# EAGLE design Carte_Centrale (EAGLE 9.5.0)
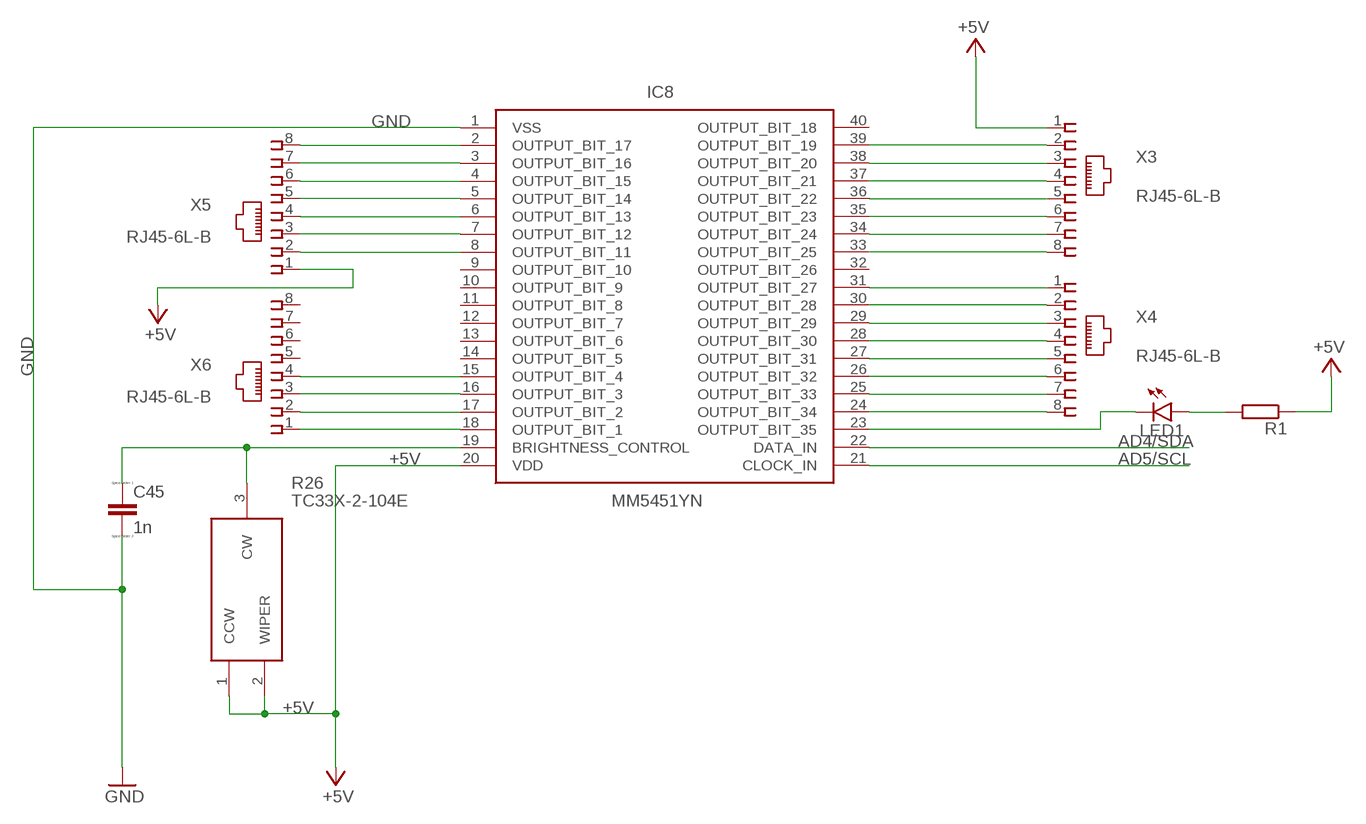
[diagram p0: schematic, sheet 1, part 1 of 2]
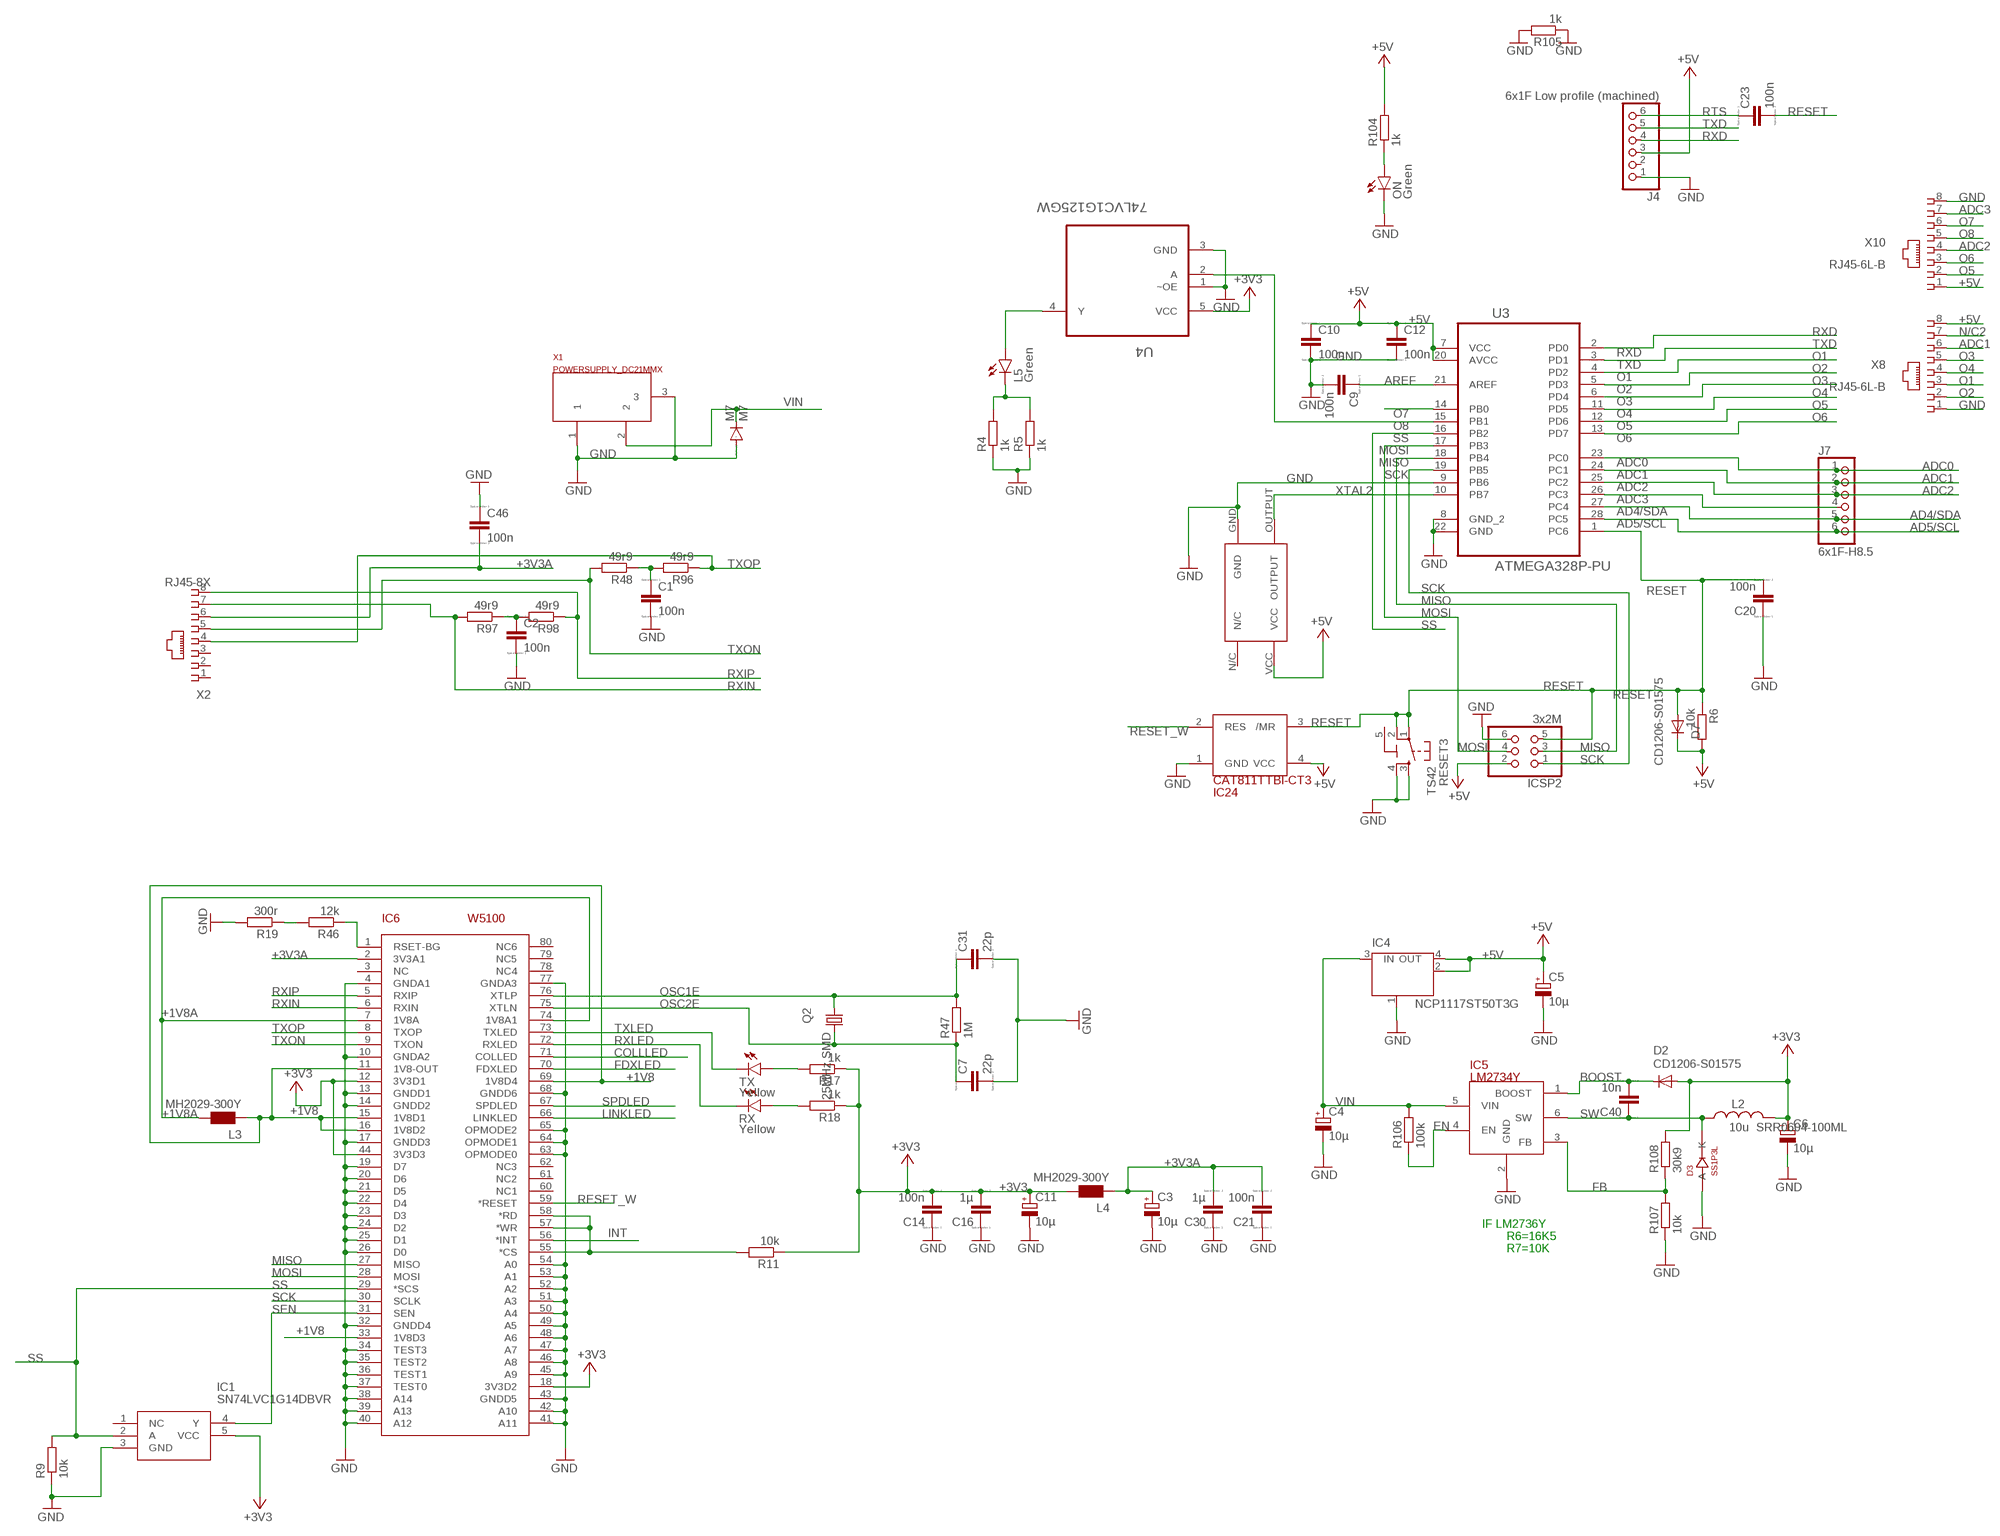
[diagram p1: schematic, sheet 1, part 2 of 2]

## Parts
C1  100n  CC2012  [C2012]
C2  100n  CC2012  [C2012]
C3  10µ  CPOL-EUE2-5  [E2-5]
C4  10µ  CPOL-EUE2-5  [E2-5]
C5  10µ  CPOL-EUE2-5  [E2-5]
C6  10µ  CPOL-EUE2-5  [E2-5]
C7  22p  CC2012  [C2012]
C9  100n  CC2012  [C2012]
C10  100n  CC2012  [C2012]
C11  10µ  CPOL-EUE2-5  [E2-5]
C12  100n  CC2012  [C2012]
C14  100n  CC2012  [C2012]
C16  1µ  CC2012  [C2012]
C20  100n  CC2012  [C2012]
C21  100n  CC2012  [C2012]
C23  100n  CC2012  [C2012]
C30  1µ  CC2012  [C2012]
C31  22p  CC2012  [C2012]
C40  10n  CC2012  [C2012]
C45  1n  CC2012  [C2012]
C46  100n  CC2012  [C2012]
D2  CD1206-S01575  DIODE-MINIMELF  [MINIMELF]
D3  SS1P3L  [DO220AAL]
D7  CD1206-S01575  DIODE-MINIMELF  [MINIMELF]
IC1  SN74LVC1G14DBVR  [SOT95P280X145-5N]
IC4  NCP1117ST50T3G  LINEAR_MC33269ST  [LINEAR_SOT223]
IC5  LM2734Y  LM2736Y  [SOT23-6]
IC6  W5100  [SQFP-S-10X10-80]
IC8  MM5451YN  [DIP1556W46P254L5207H635Q40N]
IC24  CAT811TTBI-CT3  STM812  [SOT143]
ICSP2  3x2M  PINHD-2X3  [2X03]
J4  6x1F Low profile (machined)  PINHD-1X6TH  [1X06-TH]
J7  6x1F-H8.5  PINHD-1X6  [1X06]
L2  10u SRR0604-100ML  L-USSRR0604  [SRR0604]
L3  MH2029-300Y  WE-CBF_0805  [0805]
L4  MH2029-300Y  WE-CBF_0805  [0805]
L5  Green  LEDCHIPLED_0805  [CHIPLED_0805]
LED1  LED5MM  [LED5MM]
M7  M7  1N4004  [DO41-10]
ON  Green  LEDCHIPLED_0805  [CHIPLED_0805]
Q2  25MHz SMD  CRYSTALHC49UP  [HC49UP]
R1  R-EU_0204/7  [0204/7]
R4  1k  R-EU_M0805  [M0805]
R5  1k  R-EU_M0805  [M0805]
R6  10k  R-EU_M0805  [M0805]
R9  10k  R-EU_M0805  [M0805]
R11  10k  R-EU_M0805  [M0805]
R17  1k  R-EU_M0805  [M0805]
R18  1k  R-EU_M0805  [M0805]
R19  300r  R-EU_M0805  [M0805]
R26  TC33X-2-104E  [TC33X-2]
R46  12k  R-EU_M0805  [M0805]
R47  1M  R-EU_M0805  [M0805]
R48  49r9  R-EU_M0805  [M0805]
R96  49r9  R-EU_M0805  [M0805]
R97  49r9  R-EU_M0805  [M0805]
R98  49r9  R-EU_M0805  [M0805]
R104  1k  R-EU_M0805  [M0805]
R105  1k  R-EU_M0805  [M0805]
R106  100k  R-EU_M0805  [M0805]
R107  10k  R-EU_M0805  [M0805]
R108  30k9  R-EU_M0805  [M0805]
RESET3  TS42  [TS42]
RX  Yellow  LEDCHIPLED_0805  [CHIPLED_0805]
TX  Yellow  LEDCHIPLED_0805  [CHIPLED_0805]
U3  ATMEGA328P-PU  [DIP254P762X457-28]
U4  74LVC1G125GW  [SOT65P210X110-5N]
U$1  NCT050C  [NCT050C_FOOTPRINT]
X1  POWERSUPPLY_DC21MMX  [POWERSUPPLY_DC-21MM]
X2  RJ45-8X  [RJ45-NO-SHIELD]
X3  RJ45-6L-B  [RJ45-NO-SHIELD]
X4  RJ45-6L-B  [RJ45-NO-SHIELD]
X5  RJ45-6L-B  [RJ45-NO-SHIELD]
X6  RJ45-6L-B  [RJ45-NO-SHIELD]
X8  RJ45-6L-B  [RJ45-NO-SHIELD]
X10  RJ45-6L-B  [RJ45-NO-SHIELD]

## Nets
+1V8 [power]: IC6.11(1V8-OUT) IC6.15(1V8D1) IC6.16(1V8D2) IC6.33(1V8D3) IC6.69(1V8D4) L3.1
+1V8A [power]: IC6.7(1V8A) IC6.74(1V8A1) L3.2
+3V3 [power]: C6.+ C11.+ C14.2 C16.2 D2.A IC1.5(VCC) IC6.12(3V3D1) IC6.18(3V3D2) IC6.44(3V3D3) L2.P$2 L4.2 R11.1 R17.1 R18.1 R108.2 U4.5(VCC)
+3V3A [power]: C3.+ C21.2 C30.2 C46.2 IC6.2(3V3A1) L4.1 X2.6
+5V [power]: C5.+ C10.1 C12.1 D7.C IC4.2(OUT) IC4.4(OUT) IC8.20(VDD) IC24.4(VCC) ICSP2.2 J4.3 R1.1 R6.2 R26.1(CCW) R26.2(WIPER) R104.2 U3.7(VCC) U3.20(AVCC) U$1.VCC X3.1 X5.1 X8.8 X10.1
AD4/SDA: IC8.22(DATA_IN) J7.5 U3.27(PC4)
AD5/SCL: IC8.21(CLOCK_IN) J7.6 U3.28(PC5)
ADC0: J7.1 U3.23(PC0)
ADC1: J7.2 U3.24(PC1) X8.6
ADC2: J7.3 U3.25(PC2) X10.4
ADC3: J7.4 U3.26(PC3) X10.7
AREF: C9.1 U3.21(AREF)
BOOST: C40.2 D2.C IC5.1(BOOST)
COLLLED: IC6.71(COLLED)
EN: IC5.4(EN) R106.1
FB: IC5.3(FB) R107.2 R108.1
FDXLED: IC6.70(FDXLED)
GND: C1.2 C2.2 C3.- C4.- C5.- C6.- C7.2 C9.2 C10.2 C11.- C12.2 C14.1 C16.1 C20.1 C21.1 C30.1 C31.2 C45.2 C46.1 D3.P$2(A) IC1.3(GND) IC4.1(GND/ADJ) IC5.2(GND) IC6.4(GNDA1) IC6.10(GNDA2) IC6.13(GNDD1) IC6.14(GNDD2) IC6.17(GNDD3) IC6.19(D7) IC6.20(D6) IC6.21(D5) IC6.22(D4) IC6.23(D3) IC6.24(D2) IC6.25(D1) IC6.26(D0) IC6.32(GNDD4) IC6.34(TEST3) IC6.35(TEST2) IC6.36(TEST1) IC6.37(TEST0) IC6.38(A14) IC6.39(A13) IC6.40(A12) IC6.41(A11) IC6.42(A10) IC6.43(GNDD5) IC6.45(A9) IC6.46(A8) IC6.47(A7) IC6.48(A6) IC6.49(A5) IC6.50(A4) IC6.51(A3) IC6.52(A2) IC6.53(A1) IC6.54(A0) IC6.63(OPMODE0) IC6.64(OPMODE1) IC6.65(OPMODE2) IC6.68(GNDD6) IC6.77(GNDA3) IC8.1(VSS) IC24.1(GND) ICSP2.6 J4.1 M7.A ON.C R4.1 R5.1 R9.1 R19.2 R105.1 R105.2 R107.1 RESET3.3 RESET3.4 U3.8(GND_2) U3.9(PB6) U3.22(GND) U4.1(~OE) U4.3(GND) U$1.GND X1.1 X1.3 X8.1 X10.8
INT: IC6.56(*INT)
LINKLED: IC6.66(LINKLED)
MISO: IC6.27(MISO) ICSP2.3 U3.18(PB4)
MOSI: IC6.28(MOSI) ICSP2.4 U3.17(PB3)
N$6: IC8.2(OUTPUT_BIT_17) X5.8
N$7: IC8.3(OUTPUT_BIT_16) X5.7
N$8: ON.A R104.1
N$9: R17.2 TX.A
N$10: C1.1 R48.1 R96.2
N$11: IC8.4(OUTPUT_BIT_15) X5.6
N$12: IC8.5(OUTPUT_BIT_14) X5.5
N$16: L5.A U4.4(Y)
N$17 [power]: C45.1 IC8.19(BRIGHTNESS_CONTROL) R26.3(CW)
N$20: IC8.6(OUTPUT_BIT_13) X5.4
N$21: IC8.7(OUTPUT_BIT_12) X5.3
N$22: R18.2 RX.A
N$23: IC8.8(OUTPUT_BIT_11) X5.2
N$25: LED1.A R1.2
N$29: C2.1 R97.1 R98.2
N$30: R19.1 R46.2
N$31: IC6.1(RSET-BG) R46.1
N$32: IC8.15(OUTPUT_BIT_4) X6.4
N$33: IC8.16(OUTPUT_BIT_3) X6.3
N$34: IC8.17(OUTPUT_BIT_2) X6.2
N$35: IC8.18(OUTPUT_BIT_1) X6.1
N$36: IC6.55(*CS) IC6.57(*WR) IC6.58(*RD) R11.2
N$38: IC8.39(OUTPUT_BIT_19) X3.2
N$39: IC8.38(OUTPUT_BIT_20) X3.3
N$40: IC8.37(OUTPUT_BIT_21) X3.4
N$41: IC8.36(OUTPUT_BIT_22) X3.5
N$42: IC8.35(OUTPUT_BIT_23) X3.6
N$43: IC8.34(OUTPUT_BIT_24) X3.7
N$44: IC8.33(OUTPUT_BIT_25) X3.8
N$45: IC8.31(OUTPUT_BIT_27) X4.1
N$46: IC8.30(OUTPUT_BIT_28) X4.2
N$47: IC8.29(OUTPUT_BIT_29) X4.3
N$48: IC8.28(OUTPUT_BIT_30) X4.4
N$49: IC8.27(OUTPUT_BIT_31) X4.5
N$50: IC8.26(OUTPUT_BIT_32) X4.6
N$51: IC8.25(OUTPUT_BIT_33) X4.7
N$52: IC8.24(OUTPUT_BIT_34) X4.8
N$54: L5.C R4.2 R5.2
N$55: IC8.23(OUTPUT_BIT_35) LED1.K(C)
N/C2: X8.7
O1: U3.4(PD2) X8.3
O2: U3.5(PD3) X8.2
O3: U3.6(PD4) X8.5
O4: U3.11(PD5) X8.4
O5: U3.12(PD6) X10.2
O6: U3.13(PD7) X10.3
O7: U3.14(PB0) X10.6
O8: U3.15(PB1) U4.2(A) X10.5
OSC1E: C31.1 IC6.76(XTLP) Q2.1 R47.2
OSC2E: C7.1 IC6.75(XTLN) Q2.2 R47.1
RESET: C20.2 C23.2 D7.A IC24.3(/MR) ICSP2.5 R6.1 RESET3.1 RESET3.2 U3.1(PC6)
RESET_W: IC6.59(*RESET) IC24.2(RES)
RTS: C23.1 J4.6
RXD: J4.4 U3.2(PD0)
RXIN: IC6.6(RXIN) R97.2 X2.7
RXIP: IC6.5(RXIP) R98.1 X2.8
RXLED: IC6.72(RXLED) RX.C
SCK: IC6.30(SCLK) ICSP2.1 U3.19(PB5)
SEN: IC1.4(Y) IC6.31(SEN)
SPDLED: IC6.67(SPDLED)
SS: IC1.2(A) IC6.29(*SCS) R9.2 U3.16(PB2)
SW [power]: C40.1 D3.P$1(K) IC5.6(SW) L2.P$1
TXD: J4.5 U3.3(PD1)
TXLED: IC6.73(TXLED) TX.C
TXON: IC6.9(TXON) R48.2 X2.5
TXOP: IC6.8(TXOP) R96.1 X2.4
VIN [VIN]: C4.+ IC4.3(IN) IC5.5(VIN) M7.C R106.2 X1.2
XTAL2: U3.10(PB7) U$1.OUTPUT
Unconnected: IC1.1(NC) IC6.3(NC) IC6.60(NC1) IC6.61(NC2) IC6.62(NC3) IC6.78(NC4) IC6.79(NC5) IC6.80(NC6) IC8.9(OUTPUT_BIT_10) IC8.10(OUTPUT_BIT_9) IC8.11(OUTPUT_BIT_8) IC8.12(OUTPUT_BIT_7) IC8.13(OUTPUT_BIT_6) IC8.14(OUTPUT_BIT_5) IC8.32(OUTPUT_BIT_26) IC8.40(OUTPUT_BIT_18) J4.2 U$1.N/C X2.1 X2.2 X2.3 X6.5 X6.6 X6.7 X6.8

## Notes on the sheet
- IF LM2736Y
- R6=16K5
- R7=10K

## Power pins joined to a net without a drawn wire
5-GND: RESET3.5(5-GND)

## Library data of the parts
C1 C2 C7 C9 C10 C12 C14 C16 C20 C21 C23 C30 C31 C40 C45 C46 = eagle-ltspice:C: CAPACITOR, European symbol; SPICEMODEL: NONE; SPICEPREFIX: C
C3-C6 C11 = rcl:CPOL-EU: POLARIZED CAPACITOR, European symbol; SPICEPREFIX: C
D2 D7 = diode:DIODE-: DIODE
D3 = SmartPrj:SS1P3L
IC1 = SN74LVC1G14DBVR:SN74LVC1G14DBVR: TEXAS INSTRUMENTS - SN74LVC1G14DBVR - IC, SCHMITT TRIGGER INVERTER, SMD Source: Datasheet; DESCRIPTION: TEXAS INSTRUMENTS - SN74LVC1G14DBVR - IC, SCHMITT TRIGGER INVERTER, SMD; HEIGHT: 1.45mm; MANUFACTURER_NAME: Texas Instruments; MANUFACTURER_PART_NUMBER: SN74LVC1G14DBVR; MOUSER_PART_NUMBER: 595-SN74LVC1G14DBVR; MOUSER_PRICE-STOCK: https://www.mouser.com/Search/Refine.aspx?Keyword=595-SN74LVC1G14DBVR
IC4 = SmartPrj:LINEAR_MC33269ST*: Adjustable Output Low Dropout Voltage Regulator 800 mA Source: http://www.onsemi.com/pub/Collateral/MC33269-D.PDF
IC5 = SmartPrj:LM2736Y
IC6 = SmartPrj:W5100
IC8 = SamacSys_Parts:MM5451YN: MM5451YN, LED Driver, 5-Digits, 5 V, 9 V, 40-Pin PDIP Source: Datasheet; DESCRIPTION: MM5451YN, LED Driver, 5-Digits, 5 V, 9 V, 40-Pin PDIP; HEIGHT: 6.35mm; MANUFACTURER_NAME: Micrel; MANUFACTURER_PART_NUMBER: MM5451YN; MOUSER_PART_NUMBER: 998-MM5451YN; MOUSER_PRICE-STOCK: https://www.mouser.com/Search/Refine.aspx?Keyword=998-MM5451YN
IC24 = SmartPrj:STM812
ICSP2 = SmartPrj:PINHD-2X3: PIN HEADER
J4 J7 = SmartPrj:PINHD-1X6: PIN HEADER
L2 = SmartPrj:L-US: INDUCTOR, American symbol
L3 L4 = wuerth-elektronik:WE-CBF: SMD EMI Suppression Ferrite Beads
L5 LED1 ON RX TX = led:LED: LED
M7 = diode:1N4004: DIODE
Q2 = crystal:CRYSTAL: CRYSTAL; OC_FARNELL: unknown; OC_NEWARK: unknown
R1 R4-R6 R9 R11 R17-R19 R46-R48 R96-R98 R104-R108 = rcl:R-EU_: RESISTOR, European symbol; SPICEPREFIX: R
R26 = TC33X-2-104E:TC33X-2-104E: Cermet 3mm SMT trimmer,0.1W 100k Bourns TC33 Series SMD Cermet Trimmer Resistor with Solder Pad Terminations, 100k +/-25% 1/10W +/-250ppm/C Top Adjust Source: Datasheet; ALLIED_NUMBER: 70155236; ALLIED_PRICE-STOCK: https://www.alliedelec.com/bourns-tc33x-2-104e/70155236/; DESCRIPTION: Cermet 3mm SMT trimmer,0.1W 100k Bourns TC33 Series SMD Cermet Trimmer Resistor with Solder Pad Terminations, 100k +/-25% 1/10W +/-250ppm/C Top Adjust; HEIGHT: mm; MANUFACTURER_NAME: Bourns; MANUFACTURER_PART_NUMBER: TC33X-2-104E; MOUSER_PART_NUMBER: 652-TC33X-2-104E; MOUSER_PRICE-STOCK: https://www.mouser.com/Search/Refine.aspx?Keyword=652-TC33X-2-104E; RS_PART_NUMBER: 4617258P; RS_PRICE-STOCK: http://uk.rs-online.com/web/p/products/4617258P
RESET3 = SmartPrj:TS42: TS42 Dongnan Electronics Tact switch VDC 12V - 50mA
U3 = Farnell_ATMEGA328PU:ATMEGA328P-PU: 8-bit Microcontroller with In-System Programmable Flash; MPN: ATMEGA328P-PU; OC_FARNELL: 1715487; OC_NEWARK: 68T2944; PACKAGE: PDIP-28; SUPPLIER: Atmel
U4 = Farnell_74LVC1G125GW:74LVC1G125GW: Bus buffer/line driver 3-state; MPN: 74LVC1G125GW; OC_FARNELL: 1631685; OC_NEWARK: 03P2776; PACKAGE: SOT-5; SUPPLIER: NXP
U$1 = NCT050C:NCT050C
X1 = SmartPrj:POWERSUPPLY_DC21MM
X2 = con-tycoelectronics:RJ45: CORCOM Modular RJ Jacks No Shield Source: www.tycoelectronics.com .. ENG_DS_1654001_1099_RJ_L_0507.pdf; MPN: RJ45-8X; OC_FARNELL: unknown; OC_NEWARK: 16R6101
X3-X6 X8 X10 = con-tycoelectronics:RJ45: CORCOM Modular RJ Jacks No Shield Source: www.tycoelectronics.com .. ENG_DS_1654001_1099_RJ_L_0507.pdf; MPN: RJ45-6L-B; OC_FARNELL: unknown; OC_NEWARK: 16R6090

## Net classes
0 default: width 0.152 mm, drill 0.61 mm, clearance 0.152 mm
1 power: width 0.152 mm, drill 0.61 mm, clearance 0.152 mm
2 VIN: width 0.61 mm, drill 0.61 mm, clearance 0.254 mm

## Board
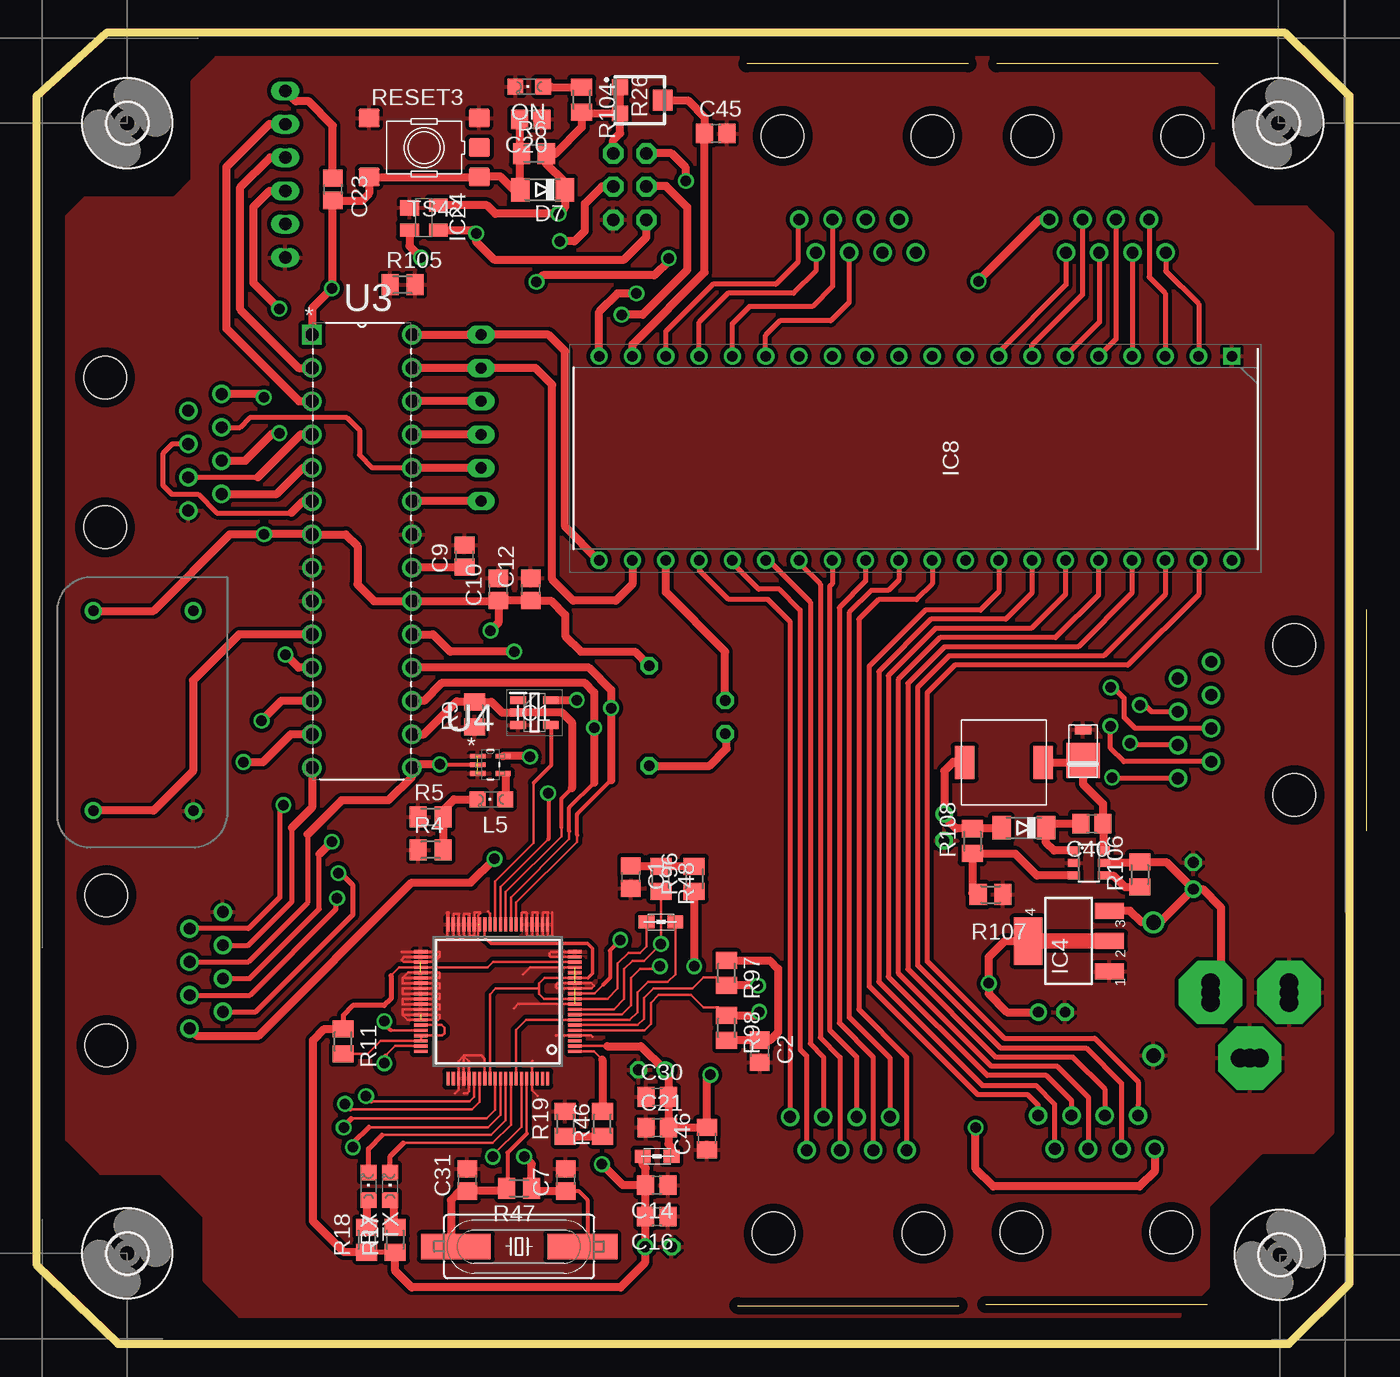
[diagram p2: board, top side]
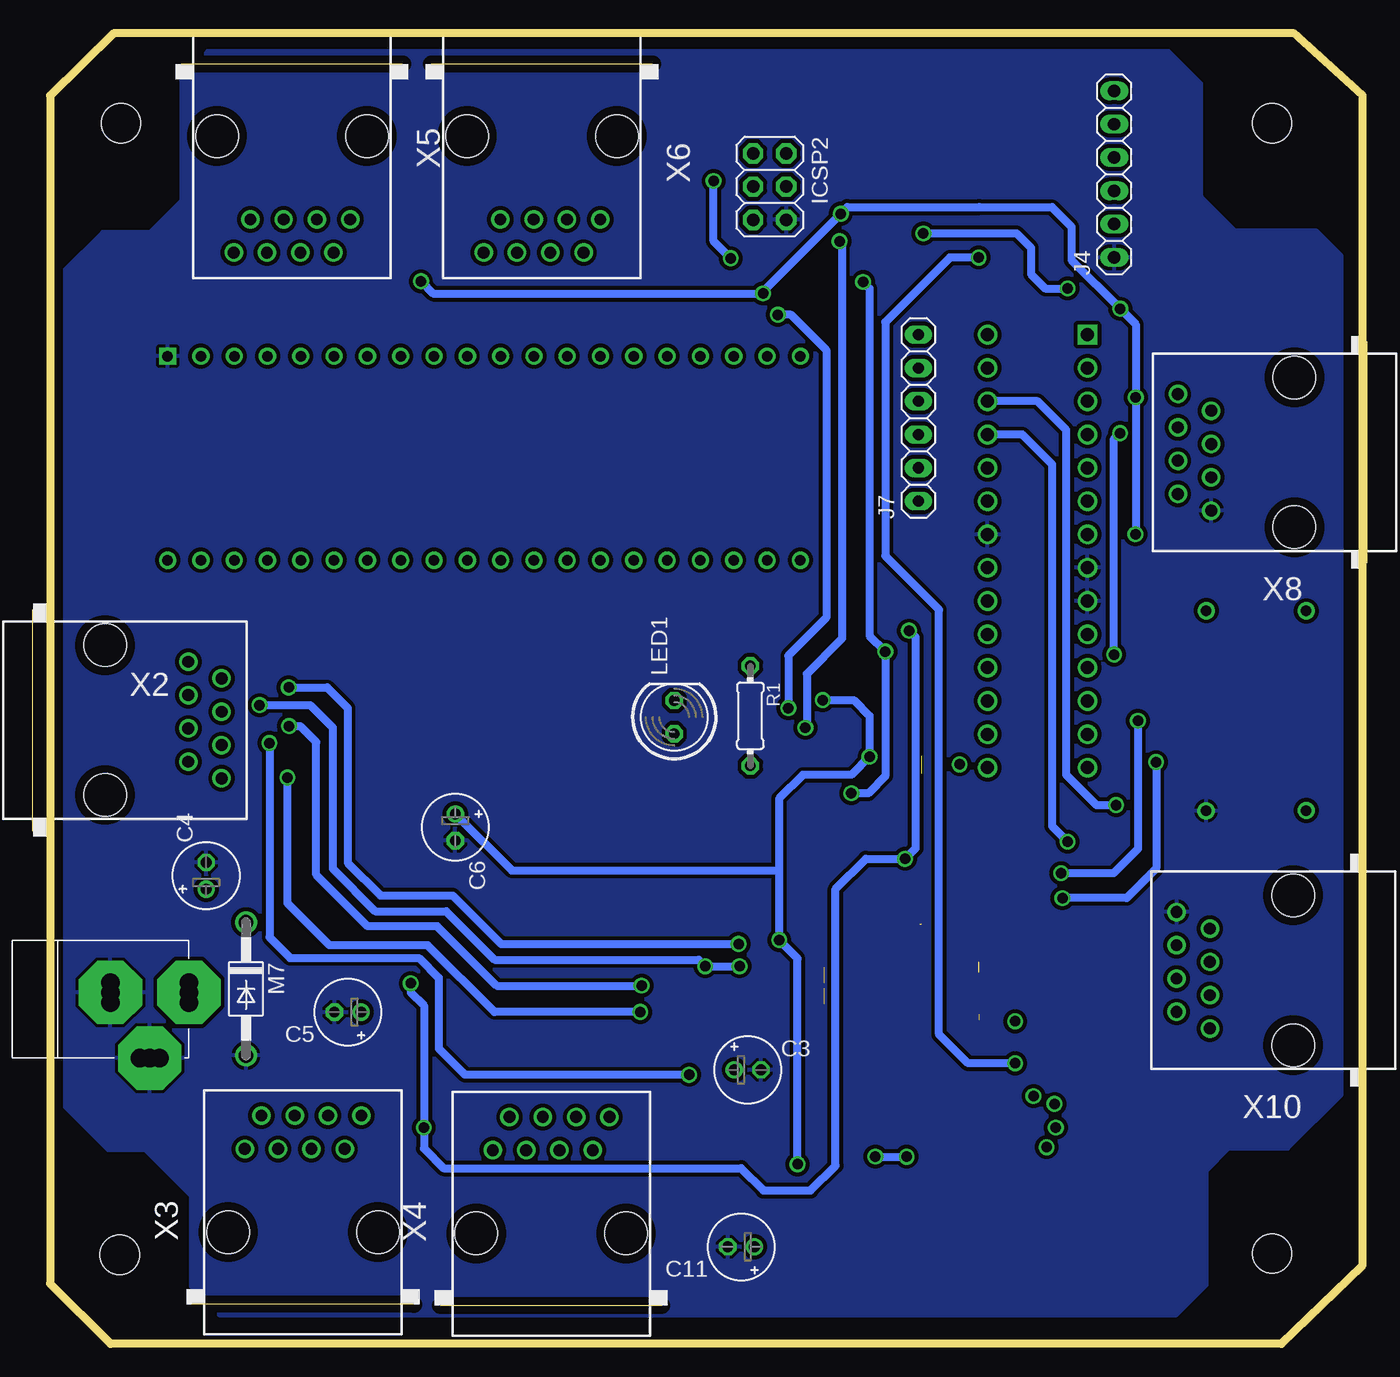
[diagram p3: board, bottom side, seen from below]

Size 101.74 x 100 mm. Coordinates in mm from the lower left corner, seen from the top.
Outline: 0.31,95.2 5.61,100 95.51,100 100.41,95.2 100.41,4.6 95.81,0 6.51,0 0.31,6 0.31,95.2
Copper layers (1*16): Top 0.035mm / dielectric 1.5mm / Bottom 0.035mm
Design rules "ArduinoETH *": minimum track width 0.2mm, minimum drill 0.8mm, track to track 0.3mm, track to pad 0.3mm, pad to pad 0.2mm, via to via 0.2mm, smd to smd 0.3mm, copper to edge 25mil, drill to drill 10mil, minimum pad ring 10mil, minimum via ring 8mil, stop-mask expansion 1mil, vias tented up to drill 30mil, thermal gap 10mil

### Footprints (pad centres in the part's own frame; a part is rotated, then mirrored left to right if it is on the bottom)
C2012 = smd 1.3 x 1.5: 1 -0.85,0; 2 0.85,0
E2-5 = drill 0.813 pad 1.27: + -1.016,0 | drill 0.813 pad 1.27 octagon: - 1.016,0
MINIMELF = smd 1.4 x 1.8: A 1.7,0; C -1.7,0
DO220AAL = smd 2.667 x 2.54: P$1 -0.7,0 | smd 0.762 x 1.27: P$2 1.65,0
SOT95P280X145-5N = smd 1.2 x 0.6: 1 -1.25,0.95; 2 -1.25,0; 3 -1.25,-0.95; 4 1.25,-0.95; 5 1.25,0.95
LINEAR_SOT223 = smd 1.219 x 2.235: 1 -2.311,-3.099; 2 0,-3.099; 3 2.311,-3.099 | smd 3.6 x 2.2: 4 0,3.099
SOT23-6 = smd 0.6 x 0.9: 1 -0.95,-1.15; 2 0,-1.15; 3 0.95,-1.15; 4 0.95,1.15; 5 0,1.15; 6 -0.95,1.15
SQFP-S-10X10-80 = smd 0.241 x 1.041: 1 -3.8,-5.879; 2 -3.4,-5.879; 3 -3,-5.879; 4 -2.6,-5.879; 5 -2.2,-5.879; 6 -1.8,-5.879; 7 -1.4,-5.879; 8 -1,-5.879; 9 -0.6,-5.879; 10 -0.2,-5.879; 11 0.2,-5.879; 12 0.6,-5.879; 13 1,-5.879; 14 1.4,-5.879; 15 1.8,-5.879; 16 2.2,-5.879; 17 2.6,-5.879; 18 3,-5.879; 19 3.4,-5.879; 20 3.8,-5.879; 41 3.8,5.879; 42 3.4,5.879; 43 3,5.879; 44 2.6,5.879; 45 2.2,5.879; 46 1.8,5.879; 47 1.4,5.879; 48 1,5.879; 49 0.6,5.879; 50 0.2,5.879; 51 -0.2,5.879; 52 -0.6,5.879; 53 -1,5.879; 54 -1.4,5.879; 55 -1.8,5.879; 56 -2.2,5.879; 57 -2.6,5.879; 58 -3,5.879; 59 -3.4,5.879; 60 -3.8,5.879 | smd 1.041 x 0.241: 21 5.879,-3.8; 22 5.879,-3.4; 23 5.879,-3; 24 5.879,-2.6; 25 5.879,-2.2; 26 5.879,-1.8; 27 5.879,-1.4; 28 5.879,-1; 29 5.879,-0.6; 30 5.879,-0.2; 31 5.879,0.2; 32 5.879,0.6; 33 5.879,1; 34 5.879,1.4; 35 5.879,1.8; 36 5.879,2.2; 37 5.879,2.6; 38 5.879,3; 39 5.879,3.4; 40 5.879,3.8; 61 -5.879,3.8; 62 -5.879,3.4; 63 -5.879,3; 64 -5.879,2.6; 65 -5.879,2.2; 66 -5.879,1.8; 67 -5.879,1.4; 68 -5.879,1; 69 -5.879,0.6; 70 -5.879,0.2; 71 -5.879,-0.2; 72 -5.879,-0.6; 73 -5.879,-1; 74 -5.879,-1.4; 75 -5.879,-1.8; 76 -5.879,-2.2; 77 -5.879,-2.6; 78 -5.879,-3; 79 -5.879,-3.4; 80 -5.879,-3.8
DIP1556W46P254L5207H635Q40N = drill 0.8 pad 1.057 square: 1 -7.779,24.13 | drill 0.8 pad 1.057: 2 -7.779,21.59; 3 -7.779,19.05; 4 -7.779,16.51; 5 -7.779,13.97; 6 -7.779,11.43; 7 -7.779,8.89; 8 -7.779,6.35; 9 -7.779,3.81; 10 -7.779,1.27; 11 -7.779,-1.27; 12 -7.779,-3.81; 13 -7.779,-6.35; 14 -7.779,-8.89; 15 -7.779,-11.43; 16 -7.779,-13.97; 17 -7.779,-16.51; 18 -7.779,-19.05; 19 -7.779,-21.59; 20 -7.779,-24.13; 21 7.779,-24.13; 22 7.779,-21.59; 23 7.779,-19.05; 24 7.779,-16.51; 25 7.779,-13.97; 26 7.779,-11.43; 27 7.779,-8.89; 28 7.779,-6.35; 29 7.779,-3.81; 30 7.779,-1.27; 31 7.779,1.27; 32 7.779,3.81; 33 7.779,6.35; 34 7.779,8.89; 35 7.779,11.43; 36 7.779,13.97; 37 7.779,16.51; 38 7.779,19.05; 39 7.779,21.59; 40 7.779,24.13
SOT143 = smd 1.2 x 1.44: 1 -0.75,-1.1 | smd 1 x 1.44: 2 0.95,-1.1; 3 0.95,1.1; 4 -0.95,1.1
2X03 = drill 0.95 pad 1.55 octagon: 1 -2.54,-1.27; 2 -2.54,1.27; 3 0,-1.27; 4 0,1.27; 5 2.54,-1.27; 6 2.54,1.27
1X06-TH = drill 0.95 pad 1.422 long: 1 -6.35,0; 2 -3.81,0; 3 -1.27,0; 4 1.27,0; 5 3.81,0; 6 6.35,0
1X06 = drill 0.85 pad 1.422 long: 1 -6.35,0; 2 -3.81,0; 3 -1.27,0; 4 1.27,0; 5 3.81,0; 6 6.35,0
SRR0604 = smd 1.5 x 2.5: P$1 3,0; P$2 -3,0
0805 = smd 1.2 x 1: 1 -1.1,0; 2 1.1,0
CHIPLED_0805 = smd 1.2 x 1.2: A 0,-1.05; C 0,1.05
LED5MM = drill 0.813 octagon: A -1.27,0; K 1.27,0
DO41-10 = drill 1.118: A 5.08,0; C -5.08,0
HC49UP = smd 5.334 x 1.93: 1 -4.826,0; 2 4.826,0
0204/7 = drill 0.813 octagon: 1 -3.81,0; 2 3.81,0
M0805 = smd 1.3 x 1.6: 1 -0.95,0; 2 0.95,0
TC33X-2 = smd 1.2 x 1.2: 1 -1,-1.625; 2 1,-1.625 | smd 1.6 x 1.5: 3 0,1.625
TS42 = smd 1.6 x 1.4: 1 -4.2,2.25; 2 4.2,2.25; 3 -4.2,-2.25; 4 4.2,-2.25; 5 -4.2,0
DIP254P762X457-28 = drill 0.991 square: 1 -7.62,33.02 | drill 0.991: 2 -7.62,30.48; 3 -7.62,27.94; 4 -7.62,25.4; 5 -7.62,22.86; 6 -7.62,20.32; 7 -7.62,17.78; 8 -7.62,15.24; 9 -7.62,12.7; 10 -7.62,10.16; 11 -7.62,7.62; 12 -7.62,5.08; 13 -7.62,2.54; 14 -7.62,0; 15 0,0; 16 0,2.54; 17 0,5.08; 18 0,7.62; 19 0,10.16; 20 0,12.7; 21 0,15.24; 22 0,17.78; 23 0,20.32; 24 0,22.86; 25 0,25.4; 26 0,27.94; 27 0,30.48; 28 0,33.02
SOT65P210X110-5N = smd 1.168 x 0.356: 1 -0.965,0.66; 2 -0.965,0; 3 -0.965,-0.66; 4 0.965,-0.66; 5 0.965,0.66
NCT050C_FOOTPRINT = drill 0.8: GND -7.44,3.74; N/C 7.82,3.73; OUTPUT -7.42,-3.89; VCC 7.81,-3.9
3,0 = hole 3: 0,0
POWERSUPPLY_DC-21MM = drill 1.4 pad 4.826 octagon: 1 -5.08,-3.353; 2 -0.076,-6.35; 3 -0.076,-0.356 | drill 1.4: 4 -5.08,-4.115; 5 -5.08,-2.591; 6 -0.838,-0.356; 7 0.686,-0.356; 8 -0.838,-6.35; 9 0.686,-6.35
RJ45-NO-SHIELD = drill 0.9 pad 1.4: 1 -4.445,6.35; 2 -3.175,8.89; 3 -1.905,6.35; 4 -0.635,8.89; 5 0.635,6.35; 6 1.905,8.89; 7 3.175,6.35; 8 4.445,8.89 | hole 3.251: -5.715,0; 5.715,0

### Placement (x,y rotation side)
C1  45.62,35.6 270 top
C2  55.46,22.32 270 top
C3  47.21,20.9 0 bottom
C4  88.51,35.7 90 bottom
C5  77.71,25.3 180 bottom
C6  69.51,39.4 270 bottom
C7  40.65,12.51 90 top
C9  32.93,60.08 90 top
C10  35.52,57.54 90 top
C11  47.71,7.4 180 bottom
C12  37.97,57.54 90 top
C14  47.6,12.11 180 top
C16  47.6,9.72 180 top
C20  37.99,93.39 180 top
C21  47.62,16.5 0 top
C23  22.88,88.06 270 top
C30  47.62,18.84 0 top
C31  33.14,12.51 90 top
C40  80.77,39.68 180 top
C45  52.09,92.32 0 top
C46  51.42,15.66 90 top
D2  75.59,39.36 180 top
D3  80.11,45.21 90 top
D7  38.88,88.03 180 top
IC1  38.26,48.14 0 top
IC4  79.01,30.72 90 top
IC5  80.55,36.67 270 top
IC6  35.47,26.12 90 top
IC8  67.33,67.55 270 top
IC24  29.83,85.9 270 top
ICSP2  45.54,88.27 270 bottom
J4  19.26,89.22 90 bottom
J7  34.19,70.63 90 bottom
L2  74.07,44.34 0 top
L3  47.91,32.17 0 top
L4  47.62,14.3 180 top
L5  34.97,41.53 90 top
LED1  52.81,47.8 90 bottom
M7  85.48,27.07 270 bottom
ON  37.86,95.89 90 top
Q2  37.09,7.43 0 top
R1  47.01,47.9 270 bottom
R4  30.34,37.69 0 top
R5  30.34,40.17 0 top
R6  38.22,90.78 0 top
R9  33.7,48.02 90 top
R11  23.67,23.07 270 top
R17  27.64,7.95 90 top
R18  25.48,7.95 90 top
R19  40.6,16.79 90 top
R26  46.42,94.85 270 top
R46  43.45,16.79 270 top
R47  37.09,11.87 180 top
R48  47.91,35.48 270 top
R96  50.45,35.48 90 top
R97  52.92,28.29 270 top
R98  52.92,24.1 270 top
R104  41.87,94.9 270 top
R105  28.21,80.78 0 top
R106  84.43,35.79 90 top
R107  73.05,34.27 180 top
R108  71.66,38.34 90 top
RESET3  29.85,91.24 180 top
RX  25.61,12.01 0 top
TX  27.26,12.01 0 top
U3  28.92,43.96 0 top
U4  34.9,44.17 0 top
U$1  8.51,48.1 90 bottom
U$2  [3,0]  95.01,93.1 0 top
U$3  [3,0]  95.11,6.8 0 top
U$6  [3,0]  7.21,6.9 0 top
U$7  [3,0]  7.21,93.1 0 top
X1  96.18,26.88 90 bottom
X2  96.23,47.58 270 bottom
X3  81.13,8.52 0 bottom
X4  62.2,8.42 0 bottom
X5  81.97,92.12 180 bottom
X6  62.9,92.12 180 bottom
X8  5.51,68 90 bottom
X10  5.61,28.5 90 bottom

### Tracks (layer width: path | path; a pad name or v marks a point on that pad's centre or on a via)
+1V8
  Top 0.2: IC6.69 34.87,26.66 35.31,27.1 38.61,27.1 | IC6.33 34.47,31.01 | IC6.15 42.35,27.92 | IC6.16 IC6.15 | 38.61,27.1 38.61,27.5 39.03,27.92 IC6.15 | 38.61,27.1 38.61,26.7 39,26.32 IC6.11 43.83,26.32 44.61,27.1 44.61,29.01 45.42,29.82 46.31,29.82 46.81,30.32 L3.1
  Top 0.254: 34.47,31.01 34.94,30.54 42.33,30.54 42.71,30.16 42.71,28.28 42.35,27.92
+1V8A
  Top 0.2: IC6.74 36.87,23.96 37.63,24.72 IC6.7 45.53,24.72 46.11,25.3 46.11,26.8 46.91,27.6 48.41,27.6 49.01,28.2 L3.2
+3V3  (via drill 0.8)
  Top 0.2: IC6.18 35.09,29.12 34.69,28.72 IC6.44 27.93,28.72 27.31,28.1 | IC6.12 42.83,26.72 43.51,27.4
  Top 0.254: D2.A 73.82,39.29 | R108.2 71.48,39.11
  Top 0.3: C11.+ 46.75,7.45 | 43.51,27.4 44.01,27.9 44.01,30 v44.81,30.8
  Top 0.305: IC1.5 | v37.92,44.79 37.92,44.83 | 46.62,12.23 C14.2
  Top 0.4: R17.1 R18.1 | 27.31,28.1 27.31,26.3 26.81,25.8 24.41,25.8 23.67,25.06 R11.1
  Top 0.6: R17.1 27.64,5.57 28.9,4.31 44.83,4.31 46.7,6.17 C11.+ | IC1.5 v41.49,49.1 | 73.82,39.29 R108.2 70.42,39.29 69.51,40.2 C6.+ 69.51,43.7 70.21,44.4 71.01,44.4 L2.P$2 | 37.92,44.83 U4.5 | C14.2 46.75,13.43 46.52,13.69 L4.2 | R18.1 23.74,7 21.37,9.37 21.37,23.16 22.23,24.02 R11.1 | 46.75,7.45 C16.2 C14.2 | C14.2 45,12.11 v43.41,13.7
  Bottom 0.6: v43.41,13.7 43.41,29.4 v44.81,30.8 44.81,36.1 | C6.+ 65.2,36.1 44.81,36.1 | v41.49,49.1 39.11,49.1 37.92,47.91 v37.92,44.79 39.31,43.4 43.01,43.4 44.81,41.6 44.81,36.1
+3V3A  (via drill 0.8)
  Top 0.2: IC6.2 43.8,22.72 43.81,22.7
  Top 0.305: C46.2
  Top 0.4: X2.6 83.84,45.67 v83.69,45.83
  Top 0.6: C21.2 C30.2 48.47,20.65 C3.+ 46.39,22.7 43.81,22.7 | C21.2 C46.2 | C21.2 48.47,15.25 48.72,15 L4.1 | v51.68,20.53 51.42,20.28 C46.2
  Bottom 0.6: v83.69,45.83 83.69,31.01 82.11,29.43 72.28,29.43 70.78,27.93 70.78,22.53 68.78,20.53 v51.68,20.53
+5V  (via drill 0.8)
  Top 0.6: C12.1 39.52,56.7 40.61,55.6 40.61,54 41.81,52.8 45.92,52.8 R1.1 | IC4.4 74.14,30.72 72.91,29.5 v72.91,27.5 72.91,26.7 74.31,25.3 C5.+ | U$1.VCC 9.21,55.91 15.05,61.75 v17.64,61.75 | 16.81,86.7 18.06,87.95 J4.3 | v17.61,72.2 17.37,72.44 X8.8 | v40.11,86.2 35.28,86.2 34.63,86.85 | R104.2 41.97,93.85 R26.2 | X10.1 12.52,23.5 17.21,23.5 28.9,35.19 33.4,35.19
  Top 0.61: R26.1 R26.2 44.79,92.33 44.27,91.81 ICSP2.2 44.11,90.81 | X5.1 76.83,85.77 72.13,81.08 v72.13,81.05 | 31.06,86.98 IC24.4 34.63,86.85 | R104.2 41.87,92.78 39.87,90.78 R6.2 39.17,90 40.58,88.59 D7.C 40.58,86.67 v40.11,86.2 | C10.1 35.48,56.66 U3.20 26.03,56.66 24.76,57.93 24.76,60.85 23.87,61.74 U3.7 21.28,61.75 v17.64,61.75 | C12.1 C10.1 | v18.79,78.95 16.81,80.93 16.81,86.7 | v46.05,80.12 44.59,80.12 43.2,78.73 IC8.20 | X3.1 85.57,13.16 84.41,12 73.26,12 71.91,13.36 v71.91,16.5 | 33.4,35.19 v35.21,37 | C10.1 35.52,55 v34.91,54.4
  Top 1.2: IC4.4 IC4.2
  Bottom 0.6: 17.61,77.77 v17.61,72.2 17.61,61.78 v17.64,61.75 | 29.54,86.7 24.01,86.7 22.51,85.2 22.51,82.67 v18.79,78.95 | v46.05,80.12 46.05,80.27 43.51,82.8
  Bottom 0.61: v46.05,80.12 71.2,80.12 v72.13,81.05 | v18.79,78.95 17.61,77.77 | v17.64,61.75 17.59,61.8 | 43.51,82.8 v40.11,86.2 39.61,86.7 29.54,86.7 | v72.91,27.5 72.91,26.8 71.91,25.8 v71.91,16.5 71.91,14.9 70.41,13.4 47.71,13.4 46.01,11.7 42.41,11.7 40.51,13.6 40.51,34.7 38.21,37 v35.21,37 34.41,37.8 34.41,53.9 v34.91,54.4
AD4/SDA
  Top 0.6: IC8.22 45.74,57.95 44.48,56.69 41.22,56.69 39.61,58.3 39.61,73.16 38.33,74.44 J7.5 U3.27
AD5/SCL
  Top 0.305: 33.11,76.98 J7.6
  Top 0.6: IC8.21 43.2,59.72 40.6,62.32 40.6,75.71 39.33,76.98 33.11,76.98 U3.28
ADC0
  Top 0.6: J7.1 U3.23
ADC1
  Top 0.4: X8.6 15.8,69.91 16.54,70.65 23.96,70.65 24.91,69.7 24.91,67.8 25.9,66.82 U3.24
  Top 0.6: J7.2 U3.24
ADC2  (via drill 0.8)
  Top 0.3: v22.81,38.3 22.91,38.3
  Top 0.4: X10.4 16.54,27.87 21.84,33.17 21.84,37.33
  Top 0.6: J7.3 U3.25 | v22.81,38.3 21.84,37.33
  Bottom 0.6: U3.25 26.27,69.36 24.01,67.1 24.01,39.5 v22.81,38.3
ADC3  (via drill 0.8)
  Top 0.4: X10.7 16.46,31.68 18.86,34.07 18.86,40.75 19.11,41 v19.11,41.1
  Top 0.6: J7.4 U3.26
  Bottom 0.6: U3.26 25.11,71.9 22.91,69.7 22.91,43.4 20.61,41.1 v19.11,41.1
AREF
  Top 0.305: U3.21 28.92,59.23
  Top 0.6: 28.92,59.23 C9.1
BOOST
  Top 0.6: C40.2 77.86,39.69 D2.C 77.29,38.23 77.89,37.62 IC5.1
COLLLED  (via drill 0.8)
  Top 0.2: IC6.71 35.67,17.46 34.74,16.53 25.64,16.53
  Top 0.4: 25.64,16.53 24.41,15.3 v24.41,15
EN
  Top 0.6: R106.1 83.29,34.84 82.41,35.72 IC5.4
FB
  Top 0.6: R107.2 71.66,34.39 R108.1 74.92,37.39 76.59,35.72 IC5.3
FDXLED  (via drill 0.8)
  Top 0.2: IC6.70 35.27,17.86 34.61,17.2 24.31,17.2
  Top 0.4: 24.31,17.2 23.71,16.6 v23.71,16.5
GND  (6 unrouted)
  Top 0.2: 38.11,21.6 38.07,21.56 IC6.77 38.07,19.34 38.51,18.9 | 39.91,23.5 39.93,23.52 IC6.4 42.6,23.52 42.71,23.4 | IC6.10 37.03,25.92 36.71,25.6 | IC6.40 31.71,32.03 31.71,32.9 31.61,32.9 31.61,30.9 32.11,30.9 32.11,32.8 32.51,32.8 32.51,31 32.91,31 32.91,32.8 33.31,32.8 33.31,31.1 33.71,31.1 33.71,32.9 34.11,32.9 34.11,32.84 33.94,32.67 33.94,31.23 | 33.94,30.9 33.94,31.23 | 33.94,31.23 33.95,31.23 33.95,32 | IC6.32 34.87,32.84 34.71,33 | IC6.26 37.27,32.86 37.31,32.9 37.61,32.9 37.71,32.8 37.71,31.07 38.11,31.07 38.11,32.9 38.51,32.9 38.51,31.07 38.91,31.07 38.91,32.9 39.31,32.9 39.31,31.07 39.61,31.07 39.61,32.9 | IC6.19 39.5,29.52 39.41,29.6 39.41,29.8 39.53,29.92 IC6.20 | 28.21,27.9 31.01,27.9 31.01,28.3 31,28.32 IC6.45 28.63,28.32 28.21,27.9 | 28.21,27.9 28.21,27.5 31.01,27.5 31.01,27.1 28.21,27.1 28.21,26.7 31.01,26.7 31.01,26.3 28.21,26.3 28.21,25.9 31.01,25.9 31.01,25.5 28.21,25.5 28.21,25.1 | 28.21,25.1 31.01,25.1 31.01,24.82 30.91,24.72 IC6.54 28.6,24.72 28.21,25.1 | 28.11,29.9 28.13,29.92 IC6.41 31,29.92 31.01,29.9 31.01,29.5 | 31.01,29.5 28.31,29.5 28.11,29.3 28.3,29.12 IC6.43 30.63,29.12 31.01,29.5 | IC6.17 37.93,28.72 37.41,28.2 | 32.87,21.94 33.27,21.54 IC6.65 33.27,19.26 33.11,19.1 32.91,19.1 | 32.87,21.96 32.87,21.94 | 32.87,21.94 IC6.64 | 32.87,21.96 32.47,21.56 IC6.63 32.47,19.36 32.21,19.1 | IC6.68 34.47,21.74 34.21,22 32.91,22 32.87,21.96 | IC6.14 40.03,27.52 39.91,27.4 39.91,27.2 40,27.12 IC6.13 42.63,27.12 42.81,27.3 42.6,27.52 IC6.14
  pour Bottom: 1.91,19 1.91,83 3.81,84.9 10.01,84.9 12.61,87.5 12.61,96.1 15.11,98.6 88.41,98.6 90.41,96.6 90.41,87.2 92.81,84.8 96.41,84.8 99.41,81.8 99.41,18.2 96.01,14.8 93.21,14.8 89.71,11.3 89.71,4.4 87.51,2.2 14.51,2.2 12.21,4.5 12.21,13.2 10.51,14.9 6.01,14.9
  pour Top: 4.01,87.4 10.81,87.4 12.21,88.8 12.21,96.3 14.01,98.1 87.71,98.1 90.01,95.8 90.01,89.8 93.11,86.7 97.11,86.7 99.11,84.7 99.11,16.1 97.61,14.6 93.71,14.6 89.61,10.5 89.61,4.3 87.41,2.1 15.81,2.1 13.11,4.8 13.11,9.7 9.81,13 5.21,13 2.61,15.6 2.61,86
INT  (via drill 0.8)
  Top 0.2: IC6.56 27.29,23.92
  Top 0.3: 27.29,23.92 26.81,24.4 v26.81,24.6
LINKLED  (via drill 0.8)
  Top 0.2: 25.81,18.5 33.31,18.5 33.67,18.86 IC6.66
  Top 0.4: 25.81,18.5 v25.41,18.9
MISO  (via drill 0.8)
  Top 0.2: IC6.27 36.87,33.66 41.51,38.3 41.51,38.8
  Top 0.3: 41.51,38.8 41.51,40.4 44.11,43
  Top 0.6: U3.18 42.42,51.58 44.11,49.88 v44.11,48.5 44.11,43 | v44.91,78.5 46.51,78.5 49.91,81.9 49.91,86.7 48.31,88.3 46.84,88.3 ICSP2.3
  Bottom 0.3: v44.91,78.5 44.92,78.5
  Bottom 0.6: v44.91,78.5 43.91,78.5 41.21,75.8 41.21,55.4 44.11,52.5 v44.11,48.5
MOSI  (via drill 0.8)
  Top 0.2: IC6.28 36.47,34.06 40.91,38.5 40.91,39.1
  Top 0.3: 40.91,39.1 40.91,40.9 42.81,42.8
  Top 0.6: U3.17 29.83,49.04 31.23,50.44 42.08,50.44 42.81,49.7 v42.81,47 42.81,42.8 | v40.21,84.1 41.31,84.1 42.11,84.9 42.11,86.97 43.41,88.27 ICSP2.4
  Bottom 0.6: v40.21,84.1 40.01,83.9 40.01,53.8 42.71,51.1 42.71,47.1 v42.81,47
N$6
  Top 0.4: X5.8 86.42,81.83 88.92,79.33 IC8.2
N$7
  Top 0.4: X5.7 85.15,81.37 86.38,80.14 IC8.3
N$8
  Top 0.6: ON.A 39.51,95.89 39.51,95.9 39.56,95.85 R104.1
N$9
  Top 0.305: 27.51,9.03 R17.2 | 27.51,10.71 TX.A
  Top 0.6: 27.51,10.71 27.51,9.03
N$10
  Top 0.305: 45.65,36.43 C1.1
  Top 0.6: R96.2 R48.1 45.65,36.43
N$11
  Top 0.4: IC8.4 83.88,75.36 X5.6
N$12
  Top 0.4: X5.5 82.61,76.63 IC8.5
N$16
  Top 0.305: U4.4 36.06,43.31 | L5.A 36.06,41.57
  Top 0.6: 36.06,43.31 36.06,41.57
N$17
  Top 0.305: 48.2,94.7 R26.3
  Top 0.6: R26.3 49.96,94.85 51.24,93.57 C45.1 51.24,81.73 45.74,76.23 IC8.19
N$20
  Top 0.4: X5.4 81.36,83.21 81.36,77.93 IC8.6
N$21
  Top 0.4: X5.3 80.07,80.02 76.22,76.17 IC8.7
N$22
  Top 0.305: 25.48,10.84 RX.A
  Top 0.6: 25.48,10.84 R18.2
N$23
  Top 0.4: X5.2 78.8,80.78 73.68,75.66 IC8.8
N$25
  Top 0.6: R1.2 51.6,44.09 52.91,45.4 52.91,46.43 LED1.A
N$29
  Top 0.305: C2.1 55.43,23.15
  Top 0.6: 55.43,23.15 R98.2 | R97.1 56.22,29.24 56.85,28.6 56.85,23.76 56.26,23.17 C2.1
N$30
  Top 0.6: R19.1 R46.2
N$31
  Top 0.2: IC6.1 42.8,22.32 43.45,21.67
  Top 0.6: 43.45,21.67 R46.1
N$32
  Top 0.4: X6.4 62.27,79.44 60.86,78.03 57,78.03 55.9,76.93 IC8.15
N$33
  Top 0.4: X6.3 61,80.66 59.46,79.13 54.66,79.13 53.36,77.83 IC8.16
N$34
  Top 0.4: X6.2 59.73,81.83 58.02,80.13 53.02,80.13 50.82,77.93 IC8.17
N$35
  Top 0.4: IC8.18 48.28,77.23 51.88,80.83 56.68,80.83 58.36,82.5 58.36,85.67 X6.1
N$36
  Top 0.2: IC6.57 29.61,23.52 | 29.61,23.52 31.23,23.52 31.41,23.7 31.41,24.1 31.2,24.32 IC6.55 | R11.2 25.52,22.11 26.52,23.12 IC6.58 29.61,23.14 29.61,23.52
  Top 0.305: 23.73,22.18 R11.2
N$38
  Top 0.3: 84.31,18.22 84.3,18.21 X3.2
  Top 0.4: IC8.39 88.92,57.17 83.52,51.77 70.32,51.77 68.2,49.65 68.2,29.21 74.1,23.31 81,23.31 84.31,20 84.31,18.22
N$39
  Top 0.4: IC8.38 86.38,57.17 81.68,52.47 69.88,52.47 67.48,50.07 67.48,28.9 73.81,22.57 80.34,22.57 83.03,19.88 X3.3
N$40
  Top 0.4: IC8.37 83.84,57.27 79.74,53.17 69.54,53.17 66.74,50.37 66.74,28.6 73.47,21.87 79.34,21.87 81.76,19.45 X3.4
N$41
  Top 0.3: 80.51,14.89 X3.5
  Top 0.4: IC8.36 81.3,57.17 78,53.87 69.2,53.87 66,50.67 66,28.3 73.13,21.17 78.14,21.17 80.51,18.8 80.51,14.89
N$42
  Top 0.4: IC8.35 78.76,57.17 76.16,54.57 68.86,54.57 65.26,50.97 65.26,28 72.79,20.47 77.31,20.47 79.22,18.56 X3.6
N$43
  Top 0.3: 77.93,14.89 X3.7
  Top 0.4: IC8.34 76.22,57.27 74.22,55.27 68.52,55.27 64.52,51.27 64.52,27.62 72.42,19.71 76.51,19.71 77.93,18.29 77.93,14.89
N$44
  Top 0.4: X3.8 76.68,18.21 75.88,19.01 72.07,19.01 63.78,27.3 63.78,51.67 68.08,55.97 72.28,55.97 73.68,57.37 IC8.33
N$45
  Top 0.4: IC8.31 68.6,57.97 67.4,56.77 64.5,56.77 63,55.27 63,25.52 66.65,21.87 X4.1
N$46
  Top 0.4: IC8.30 66.06,58.27 65.26,57.47 63.96,57.47 62.26,55.77 62.26,24.93 65.38,21.81 X4.2
N$47
  Top 0.4: IC8.29 63.52,58.17 61.51,56.16 61.51,24.47 64.11,21.87 X4.3
N$48
  Top 0.4: IC8.28 60.98,57.97 60.78,57.77 60.78,23.97 62.84,21.91 X4.4
N$49
  Top 0.4: X4.5 61.57,21.87 60.07,23.37 60.07,57.94 58.44,59.57 IC8.27
N$50
  Top 0.4: X4.6 60.3,21.91 59.3,22.91 59.3,56.57 56.1,59.77 IC8.26
N$51
  Top 0.4: IC8.25 53.36,59.57 55.36,57.57 56.94,57.57 58.53,55.98 58.53,22.47 59.03,21.97 X4.7
N$52
  Top 0.4: IC8.24 50.82,59.03 53.07,56.78 56.07,56.78 57.76,55.09 X4.8
N$54
  Top 0.6: R4.2 R5.2 31.29,40.7 32.12,41.53 L5.C
N$55
  Top 0.6: LED1.K 52.81,52.8 48.28,57.33 IC8.23
O1
  Top 0.4: X8.3 17.17,66.09
  Top 0.6: U3.4 20.43,69.36 17.17,66.09
O2
  Top 0.6: X8.2 18.6,64.83 20.59,66.82 U3.5
O3
  Top 0.4: X8.5 10.65,68.64 9.91,67.9 9.91,65.5 10.61,64.8 12.61,64.8 14.03,63.38 19.71,63.38
  Top 0.6: 19.71,63.38 20.6,64.28 U3.6
O4  (via drill 0.8)
  Top 0.6: U3.11 20.26,51.58 v19.27,52.57 | v18.81,69.47 18.31,69.47 16.21,67.36 X8.4
  Bottom 0.6: v18.81,69.47 19.31,68.97 19.31,52.62 v19.27,52.57
O5  (via drill 0.8)
  Top 0.4: X10.2 17,25.32 24.41,32.73 24.41,35 23.51,35.9 v23.31,35.9
  Top 0.6: U3.12 18.96,49.04 v17.45,47.53
  Bottom 0.6: v17.45,47.53 17.45,37.76 19.31,35.9 v23.31,35.9
O6  (via drill 0.8)
  Top 0.4: X10.3 16.56,26.6 23.11,33.14 23.11,33.9 v23.21,34
  Top 0.6: U3.13 19.69,46.5 17.56,44.37 v16.06,44.37
  Bottom 0.6: v16.06,44.37 16.06,36.25 18.31,34 v23.21,34
O7
  Top 0.4: X10.6 16.44,30.41 19.77,33.74 19.77,39.38
  Top 0.6: U3.14 21.3,40.91 19.77,39.38
O8  (via drill 0.8)
  Top 0.305: U4.2 31.08,44.17 v31.05,44.2
  Top 0.4: 20.96,38.86 20.96,33.63 16.46,29.14 X10.5
  Top 0.6: v31.05,44.2 29.17,44.2 U3.15 28.92,43.26 27.12,41.46 23.55,41.46 20.96,38.86
OSC1E
  Top 0.2: IC6.76 37.67,16.04
  Top 0.3: 37.67,16.04 36.21,14.58 36.21,11.94 R47.2
  Top 0.305: 32.23,7.47 Q2.1 31.89,7.81 | R47.2 36.37,12.1 | C31.1 32.56,11.66
  Top 0.6: R47.2 35.93,11.66 C31.1 | 32.56,11.66 31.89,10.98 31.89,7.81
OSC2E  (via drill 0.8)
  Top 0.2: IC6.75 37.27,16.57 35.09,14.38
  Top 0.254: 35.09,14.38 v35.09,14.27
  Top 0.305: 38.17,12 R47.1 38.26,11.66 | 41.96,7.47 Q2.2 42.3,7.81 42.3,10.98 41.63,11.66 C7.1
  Top 0.6: R47.1 38.04,13.72 v37.47,14.29 | 38.26,11.66 C7.1
  Bottom 0.3: v37.47,14.29 37.46,14.27
  Bottom 0.6: 37.46,14.27 v35.09,14.27
RESET  (via drill 0.8)
  Top 0.3: 25.63,88.97 RESET3.2
  Top 0.305: D7.A 37.17,88.04 | 37.17,93.36 C20.2
  Top 0.6: U3.1 21.3,78.99 v22.81,80.5 22.84,80.53 22.84,87.17 | C20.2 37.14,90.9 R6.1 37.18,90.69 D7.A 36.68,88.03 35.68,89.03 34.09,89.03 RESET3.1 RESET3.2 25.65,87.74 25.08,87.17 22.84,87.17 | C23.2 22.84,87.17 | ICSP2.5 46.81,84.4 45.11,82.7 35.18,82.7 33.81,84.07 v33.81,84.7 33.56,84.95 IC24.3
  Bottom 0.6: v33.81,84.7 26.71,84.7 25.61,83.6 25.61,81.6 24.51,80.5 v22.81,80.5
RESET_W  (via drill 0.8)
  Top 0.2: 26.91,22 27.63,22.72 IC6.59
  Top 0.3: 26.91,22 26.81,21.9 v26.81,21.4
  Top 0.6: IC24.2 28.73,83.73 v29.6,82.86
  Bottom 0.6: v26.81,21.4 30.41,21.4 32.61,23.6 32.61,56 36.71,60.1 36.71,77.95 31.8,82.86 v29.6,82.86
RTS
  Top 0.6: C23.1 22.88,92.93 21.04,94.77 20.06,94.77 J4.6
RXD
  Top 0.6: U3.2 20.28,74.44 15.82,78.89 15.82,88.21 18.1,90.49 J4.4
RXIN  (via drill 0.8)
  Top 0.2: R97.2 52.32,27.94 51.15,27.94 50.31,27.1 47.33,27.1 46.61,26.38 46.61,24.8 46.13,24.32 IC6.6
  Top 0.4: X2.7 83.21,44.4 82.19,45.42 v82.19,47.12
  Top 0.6: v55.3,27.32 55.28,27.34 R97.2
  Bottom 0.6: v55.3,27.32 66.36,27.32 70.88,31.84 76.18,31.84 80.11,35.77 80.11,45.9 81.33,47.12 v82.19,47.12
RXIP  (via drill 0.8)
  Top 0.2: IC6.5 46.65,23.92 47.15,24.42 47.15,26.02 47.73,26.6 50.21,26.6 51.16,25.65 52.32,25.65 R98.1
  Top 0.305: 52.6,25.37 R98.1
  Top 0.4: X2.8 82.38,43.13 v82.32,43.2
  Top 0.6: R98.1 55.14,25.05 v55.4,25.31
  Bottom 0.6: v55.4,25.31 66.53,25.31 71.61,30.4 79.11,30.4 82.32,33.61 v82.32,43.2
RXLED
  Top 0.2: IC6.72 36.07,17.06 34.94,15.93 26.64,15.93
  Top 0.4: RX.C 25.61,14.89 26.64,15.93
SCK  (via drill 0.8)
  Top 0.2: IC6.30 35.67,34.86 39.32,38.51
  Top 0.3: v39.31,42 v39.32,41.99 39.32,38.51
  Top 0.6: U3.19 30.52,54.12 31.84,52.8 v36.71,52.8 | v48.51,82.8 48.51,82.6 47.41,81.5 38.91,81.5 v38.41,81 | ICSP2.1 48.71,90.8 49.81,89.7 v49.81,88.7
  Bottom 0.6: v39.31,42 38.01,42 36.71,43.3 v36.71,52.8 37.91,54 37.91,80.5 v38.41,81 | v48.51,82.8 49.81,84.1 v49.81,88.7
SEN
  Top 0.2: 38.21,42.8 38.21,38.2 35.27,35.26 IC6.31
  Top 0.3: IC1.4 39.51,44.1 38.21,42.8
SPDLED  (via drill 0.8)
  Top 0.2: IC6.67 34.07,18.46 33.51,17.9 24.21,17.9
  Top 0.4: 24.21,17.9 v23.81,18.3
SS
  Top 0.2: IC6.29 36.07,34.46 40.31,38.7 40.31,39.4
  Top 0.3: 40.31,39.4 40.31,41.6 41.11,42.4
  Top 0.305: 33.7,49 R9.2
  Top 0.6: R9.2 34.99,48.97 35.81,48.14 IC1.2 40.37,48.14 41.11,47.4 41.11,42.4 | U3.16 29.82,46.5 32.33,49 33.7,49
SW
  Top 0.254: D3.P$1 80.22,44.51
  Top 0.3: 79.93,44.34 D3.P$1
  Top 0.6: L2.P$1 79.93,44.34 | D3.P$1 80.11,42.7 81.62,41.19 C40.1 81.7,39.6 IC5.6
TXD
  Top 0.6: U3.3 20.32,71.9 14.78,77.43 14.78,89.77 18.04,93.03 J4.5
TXLED
  Top 0.2: IC6.73 36.47,16.71 35.09,15.32 28.26,15.32
  Top 0.4: TX.C 27.26,14.32 28.26,15.32
TXON  (via drill 0.8)
  Top 0.2: IC6.9 44.33,25.52 45.11,26.3 45.11,28.6 45.73,29.22 46.63,29.22 v47.91,30.5 R48.2
  Top 0.4: X2.5 84.09,46.94 83.22,47.81 83.22,49.27 82.42,50.07 v82.22,50.07
  Bottom 0.6: v82.22,50.07 79.28,50.07 77.71,48.5 77.71,36.7 75.21,34.2 69.71,34.2 66.01,30.5 v47.91,30.5
TXOP  (via drill 0.8)
  Top 0.2: IC6.8 44.93,25.12 45.61,25.8 45.61,27.9 46.33,28.62 47.65,28.62
  Top 0.254: 47.65,28.62 v47.83,28.8
  Top 0.4: X2.4 85.34,48.21 84.83,48.72 v84.44,48.72
  Top 0.6: R96.1 v50.45,28.8
  Bottom 0.6: v47.83,28.8 v50.45,28.8 50.95,29.3 66.51,29.3 70.21,33 75.61,33 78.86,36.25 78.86,47 80.58,48.72 v84.44,48.72
VIN
  Top 0.61: IC5.5 84.36,36.67 R106.2 86.45,36.74 C4.+ | C4.+ 85.98,32.15 M7.C 84.58,32.15 83.69,33.03 IC4.3 | C4.+ 89.23,34.68 90.63,33.28 90.63,27.6 X1.2
XTAL2
  Top 0.6: U3.10 15.73,54.12 12.22,50.61 12.22,43.68 9.22,40.68 U$1.OUTPUT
